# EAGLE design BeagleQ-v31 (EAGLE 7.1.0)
BOARD_NUMBER: 1.0
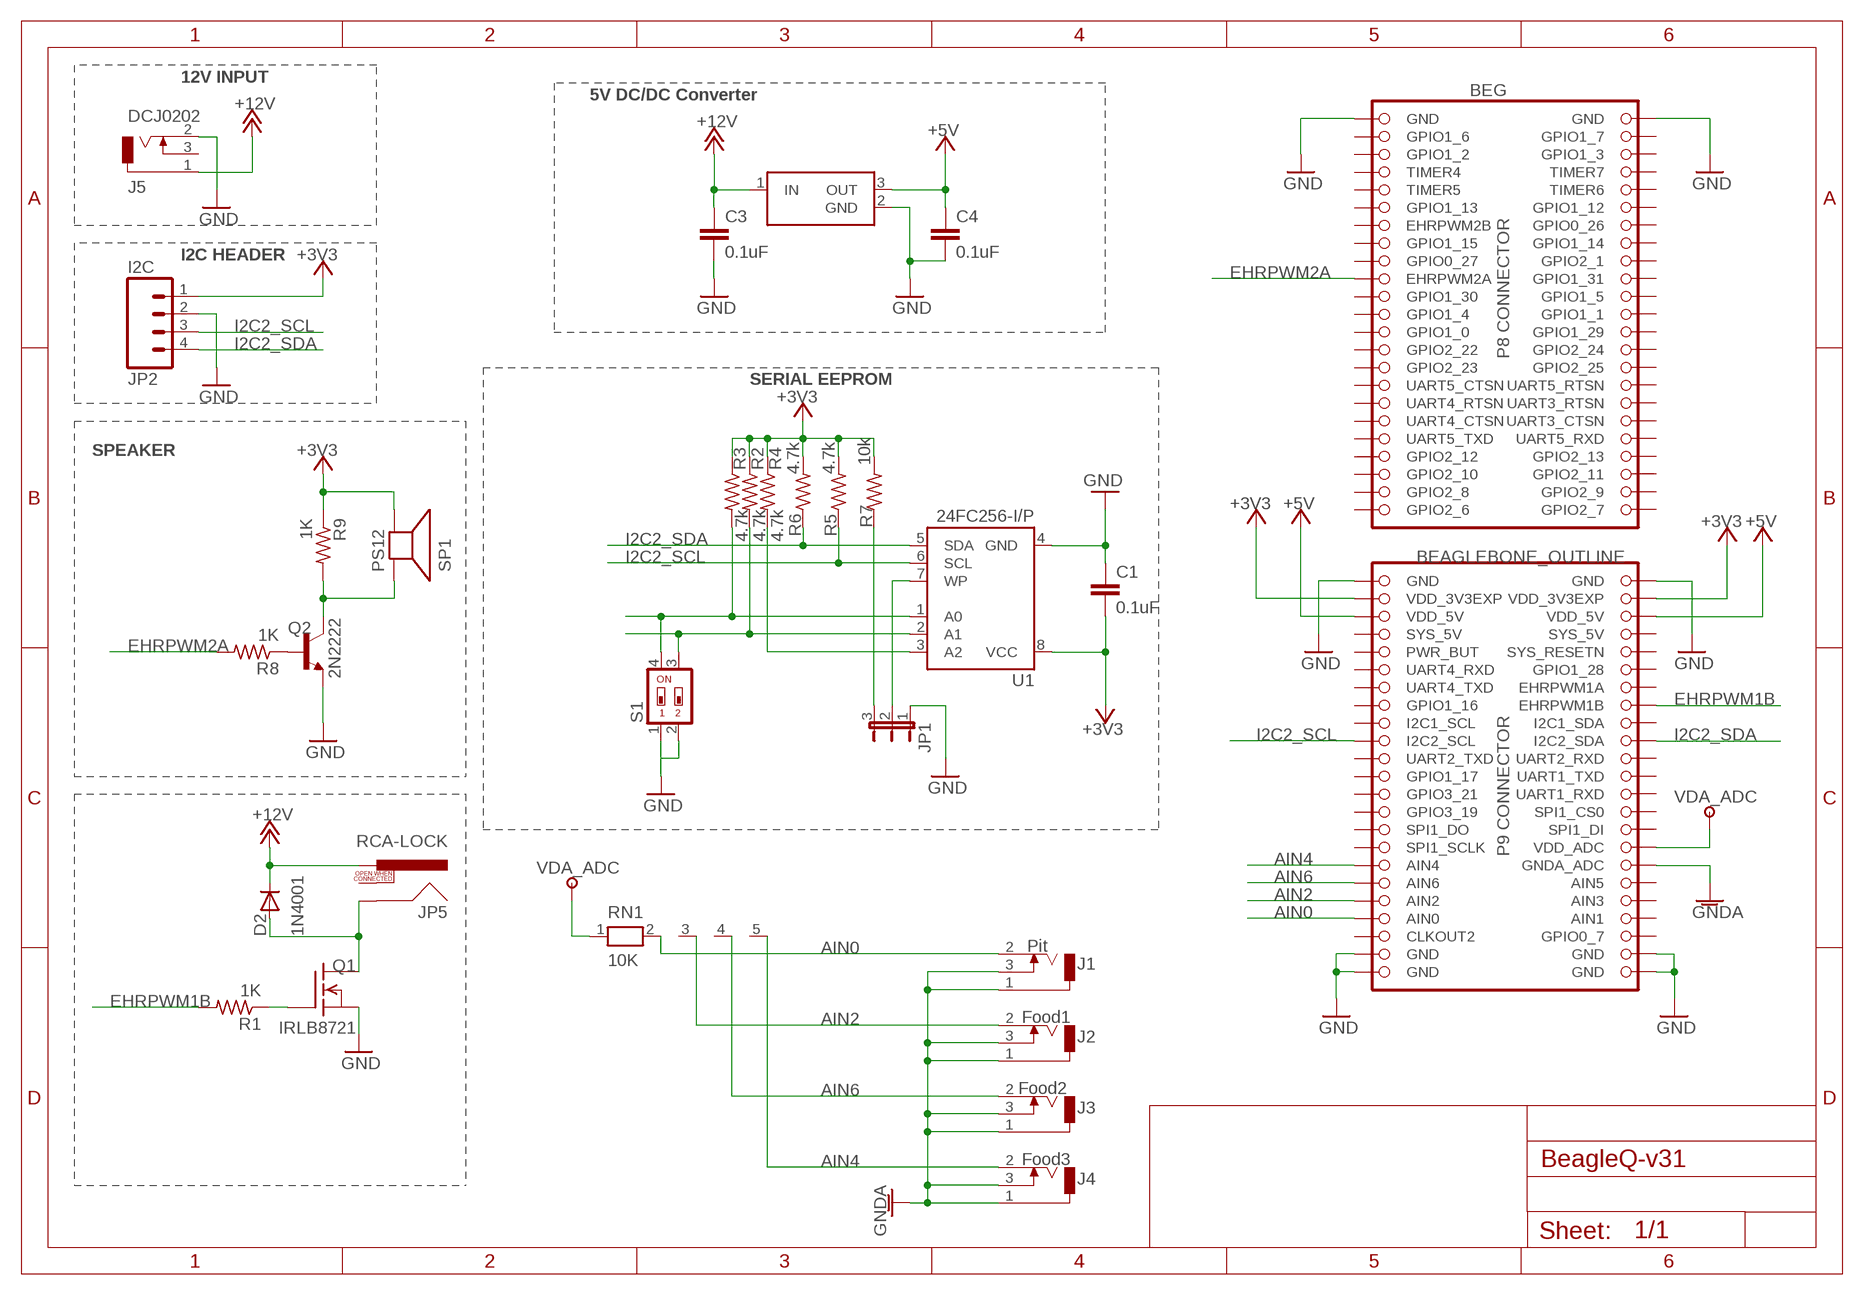
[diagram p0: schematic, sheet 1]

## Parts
BEG  BEAGLEBONE_OUTLINE  [BEAGLEBONE_SHIELD]
C1  0.1uF  C2.5/2  [C2.5-2]
C3  0.1uF  C2.5/2  [C2.5-2]
C4  0.1uF  C2.5/2  [C2.5-2]
D2  1N4001  1N4004  [DO41-10]
J1  Pit  MJ-2508N  [MJ-2508N]
J2  Food1  MJ-2508N  [MJ-2508N]
J3  Food2  MJ-2508N  [MJ-2508N]
J4  Food3  MJ-2508N  [MJ-2508N]
J5  DCJ0202  [DCJ0202]
JP1  WP  JP2E  [JP2]
JP2  I2C  M04PTH  [1X04]
JP5  RCA-LOCK  [RCA_LOCK]
Q1  IRLB8721  BUZ10  [TO220]
Q2  2N2222  [TO-92]
R1  1K  R-US_0207/10  [0207/10]
R2  4.7k  R-US_0207/10  [0207/10]
R3  4.7k  R-US_0207/10  [0207/10]
R4  4.7k  R-US_0207/10  [0207/10]
R5  4.7k  R-US_0207/10  [0207/10]
R6  4.7k  R-US_0207/10  [0207/10]
R7  10k  R-US_0207/10  [0207/10]
R8  1K  R-US_0207/10  [0207/10]
R9  1K  R-US_0207/10  [0207/10]
RN1  10K  RN04  [RN-5]
S1  SWS002  [SMS-002]
SP1  PS12  SPEAKER/PS12  [PS12]
U1  24FC256-I/P  AT24CP  [DIL08]
U2  OKI-78SRHZNTL  [OKI-78SR-HZNTL]

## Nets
+3V3: BEG.49(VDD_3V3EXP) BEG.50(VDD_3V3EXP) C1.2 JP2.1 R2.1 R3.1 R4.1 R5.2 R6.2 R7.2 R9.1 SP1.P$2(-) U1.8(VCC)
+5V [VDD]: BEG.51(VDD_5V) BEG.52(VDD_5V) C4.1 U2.3(OUT)
+12V: C3.1 D2.C J5.1 JP5.PIN U2.1(IN)
AIN0: BEG.85(AIN0) J1.2 RN1.2
AIN2: BEG.83(AIN2) J2.2 RN1.3
AIN4: BEG.79(AIN4) J4.2 RN1.5
AIN6: BEG.81(AIN6) J3.2 RN1.4
BLOWER_L [VCC_12V]: D2.A JP5.SHELL Q1.2(D)
EHRPWM1B: BEG.62(EHRPWM1B) R1.2
EHRPWM2A: BEG.19(EHRPWM2A) R8.2
GND [GND]: BEG.1(GND) BEG.2(GND) BEG.47(GND) BEG.48(GND) BEG.89(GND) BEG.90(GND) BEG.91(GND) BEG.92(GND) C1.1 C3.2 C4.2 J5.2 JP1.1 JP2.2 Q1.3(S) Q1.4(S) Q2.1(E) S1.1 S1.2 U1.4(GND) U2.2(GND)
GNDA: BEG.80(GNDA_ADC) J1.1 J1.3 J2.1 J2.3 J3.1 J3.3 J4.1 J4.3
I2C2_SCL: BEG.65(I2C2_SCL) JP2.3 R5.1 U1.6(SCL)
I2C2_SDA: BEG.66(I2C2_SDA) JP2.4 R6.1 U1.5(SDA)
N$1: R2.2 S1.3 U1.2(A1)
N$2: R3.2 S1.4 U1.1(A0)
N$3: JP1.2 U1.7(WP)
N$4: Q1.1(G) R1.1
N$5: JP1.3 R7.1
N$9: R4.2 U1.3(A2)
N$12: Q2.2(B) R8.1
N$13: Q2.3(C) R9.2 SP1.P$1(+)
VDA_ADC: BEG.78(VDD_ADC) RN1.1
Unconnected: BEG.3(GPIO1_6) BEG.4(GPIO1_7) BEG.5(GPIO1_2) BEG.6(GPIO1_3) BEG.7(TIMER4) BEG.8(TIMER7) BEG.9(TIMER5) BEG.10(TIMER6) BEG.11(GPIO1_13) BEG.12(GPIO1_12) BEG.13(EHRPWM2B) BEG.14(GPIO0_26) BEG.15(GPIO1_15) BEG.16(GPIO1_14) BEG.17(GPIO0_27) BEG.18(GPIO2_1) BEG.20(GPIO1_31) BEG.21(GPIO1_30) BEG.22(GPIO1_5) BEG.23(GPIO1_4) BEG.24(GPIO1_1) BEG.25(GPIO1_0) BEG.26(GPIO1_29) BEG.27(GPIO2_22) BEG.28(GPIO2_24) BEG.29(GPIO2_23) BEG.30(GPIO2_25) BEG.31(UART5_CTSN) BEG.32(UART5_RTSN) BEG.33(UART4_RTSN) BEG.34(UART3_RTSN) BEG.35(UART4_CTSN) BEG.36(UART3_CTSN) BEG.37(UART5_TXD) BEG.38(UART5_RXD) BEG.39(GPIO2_12) BEG.40(GPIO2_13) BEG.41(GPIO2_10) BEG.42(GPIO2_11) BEG.43(GPIO2_8) BEG.44(GPIO2_9) BEG.45(GPIO2_6) BEG.46(GPIO2_7) BEG.54(SYS_5V) BEG.55(PWR_BUT) BEG.56(SYS_RESETN) BEG.57(UART4_RXD) BEG.58(GPIO1_28) BEG.59(UART4_TXD) BEG.60(EHRPWM1A) BEG.61(GPIO1_16) BEG.63(I2C1_SCL) BEG.64(I2C1_SDA) BEG.67(UART2_TXD) BEG.68(UART2_RXD) BEG.69(GPIO1_17) BEG.70(UART1_TXD) BEG.71(GPIO3_21) BEG.72(UART1_RXD) BEG.73(GPIO3_19) BEG.74(SPI1_CS0) BEG.75(SPI1_DO) BEG.76(SPI1_DI) BEG.77(SPI1_SCLK) BEG.82(AIN5) BEG.84(AIN3) BEG.86(AIN1) BEG.87(CLKOUT2) BEG.88(GPIO0_7) J5.3 JP5.SWITCH

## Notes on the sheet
- 12V INPUT
- 5V DC/DC Converter
- I2C HEADER
- SERIAL EEPROM
- SPEAKER

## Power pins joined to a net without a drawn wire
SYS_5V: BEG.53(SYS_5V)

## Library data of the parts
BEG = BeagleQ-v03:BEAGLEBONE_OUTLINE: Should match A3 pinout - but not completely tested
C1 C3 C4 = capacitor-wima:C: CAPACITOR
D2 = BeagleQ-v03:1N4004: DIODE
J1-J4 = BeagleQ-v03:MJ-2508N
J5 = BeagleQ-v03:DCJ0202: DC POWER JACK Source: DCJ0202.pdf; OC_FARNELL: unknown; OC_NEWARK: unknown
JP1 = jumper:JP2E: JUMPER
JP2 = SparkFun-Connectors:M04: Header 4 Standard 4-pin 0.1" header. Use with straight break away headers (SKU : PRT-00116), right angle break away headers (PRT-00553), swiss pins (PRT-00743), machine pins (PRT-00117), and female headers (PRT-00115). Molex polarized connector foot print use with SKU : PRT-08231 with associated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
JP5 = BeagleQ-v03:RCA
Q1 = BeagleQ-v03:BUZ10: N-Channel Enhancement MOSFET 50V; 20A; 0,080Ohm
Q2 = BeagleQ-v03:2N2222*: NPN Transistor
R1 R8 R9 = BeagleQ-v03:R-US_: RESISTOR, American symbol
R2-R7 = resistor:R-US_: RESISTOR, American symbol
RN1 = BeagleQ-v03:RN04: RESISTOR NETWORK; OC_FARNELL: unknown; OC_NEWARK: unknown
S1 = BeagleQ-v03:SWS002: SMD Dip Switch 2 pol.
SP1 = adafruit:SPEAKER: SPEAKER
U1 = BeagleQ-v03:AT24C*: 2-wire serial EEPROM; MPN: AT24C1024BW-SH-B; OC_FARNELL: 1362646; OC_NEWARK: 03P2044
U2 = BeagleQ-v03:OKI-78SR

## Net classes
0 default: width 0.203 mm
1 VCC_12V: width 0.305 mm, drill 0.406 mm
2 VDD: width 0.305 mm, drill 0.406 mm
3 GND: width 0.254 mm, drill 0.406 mm

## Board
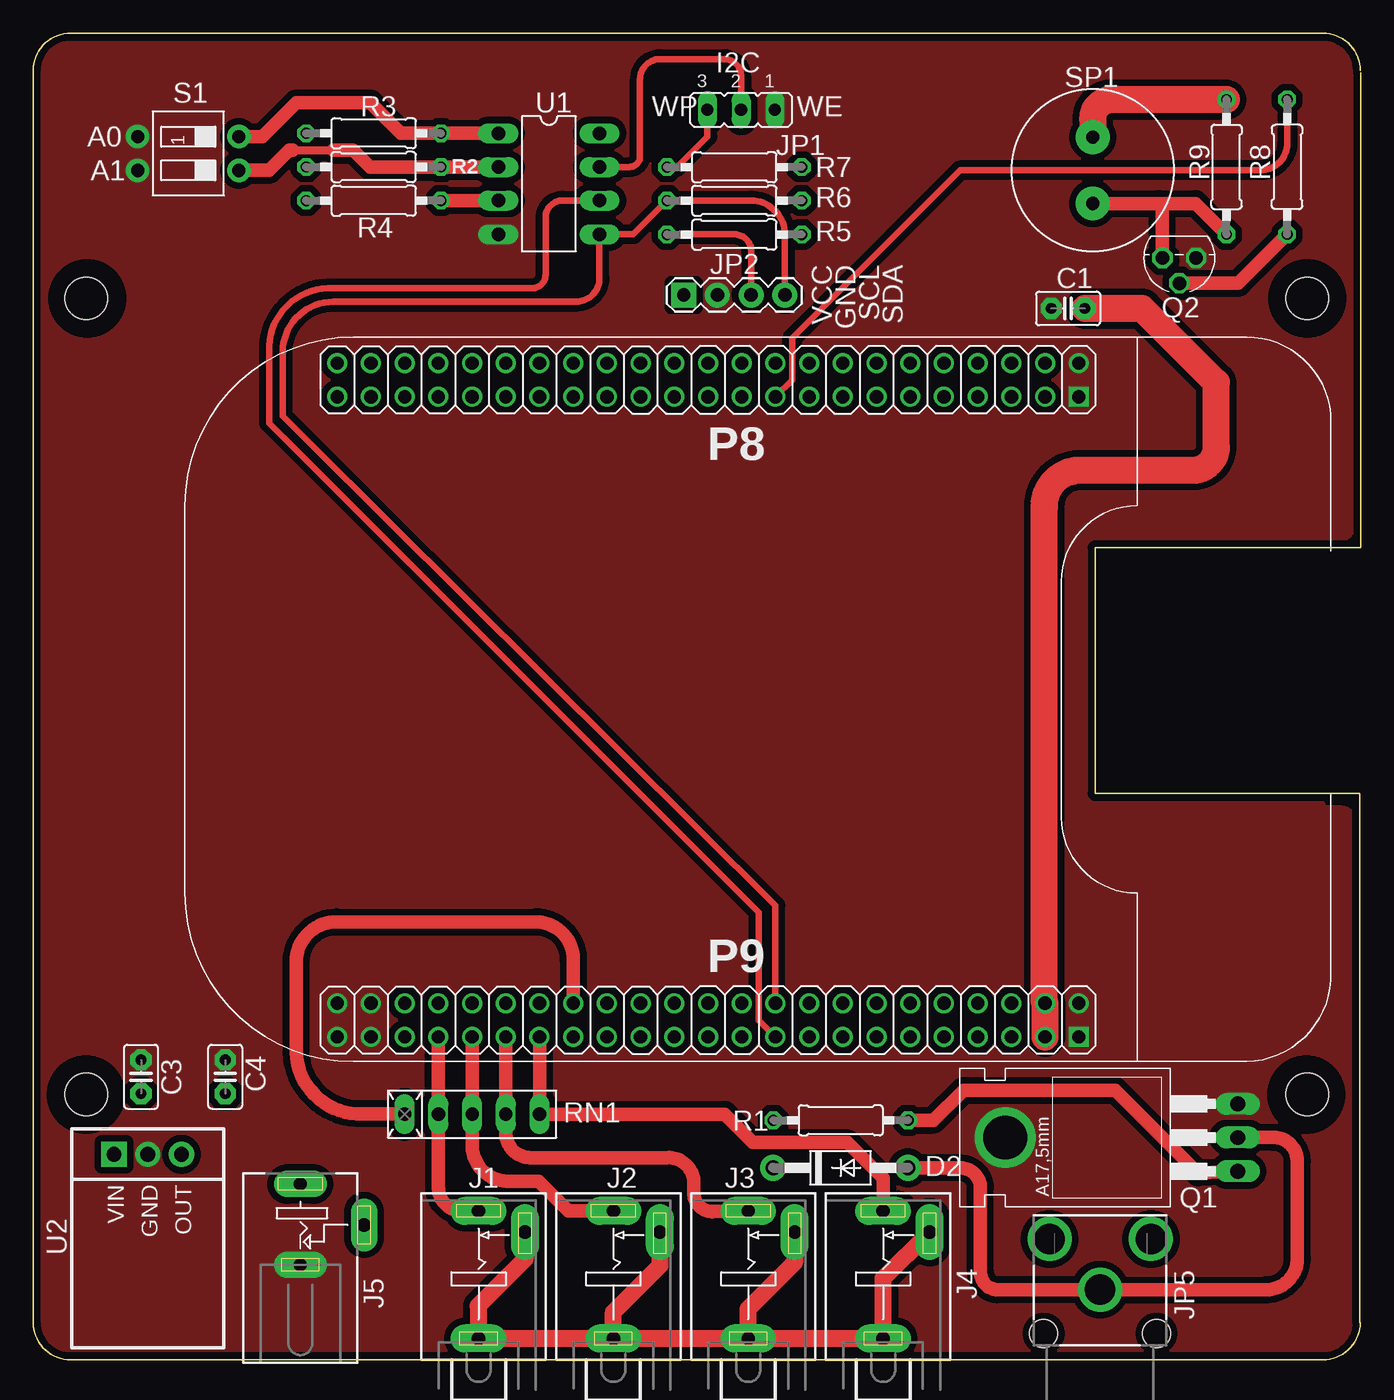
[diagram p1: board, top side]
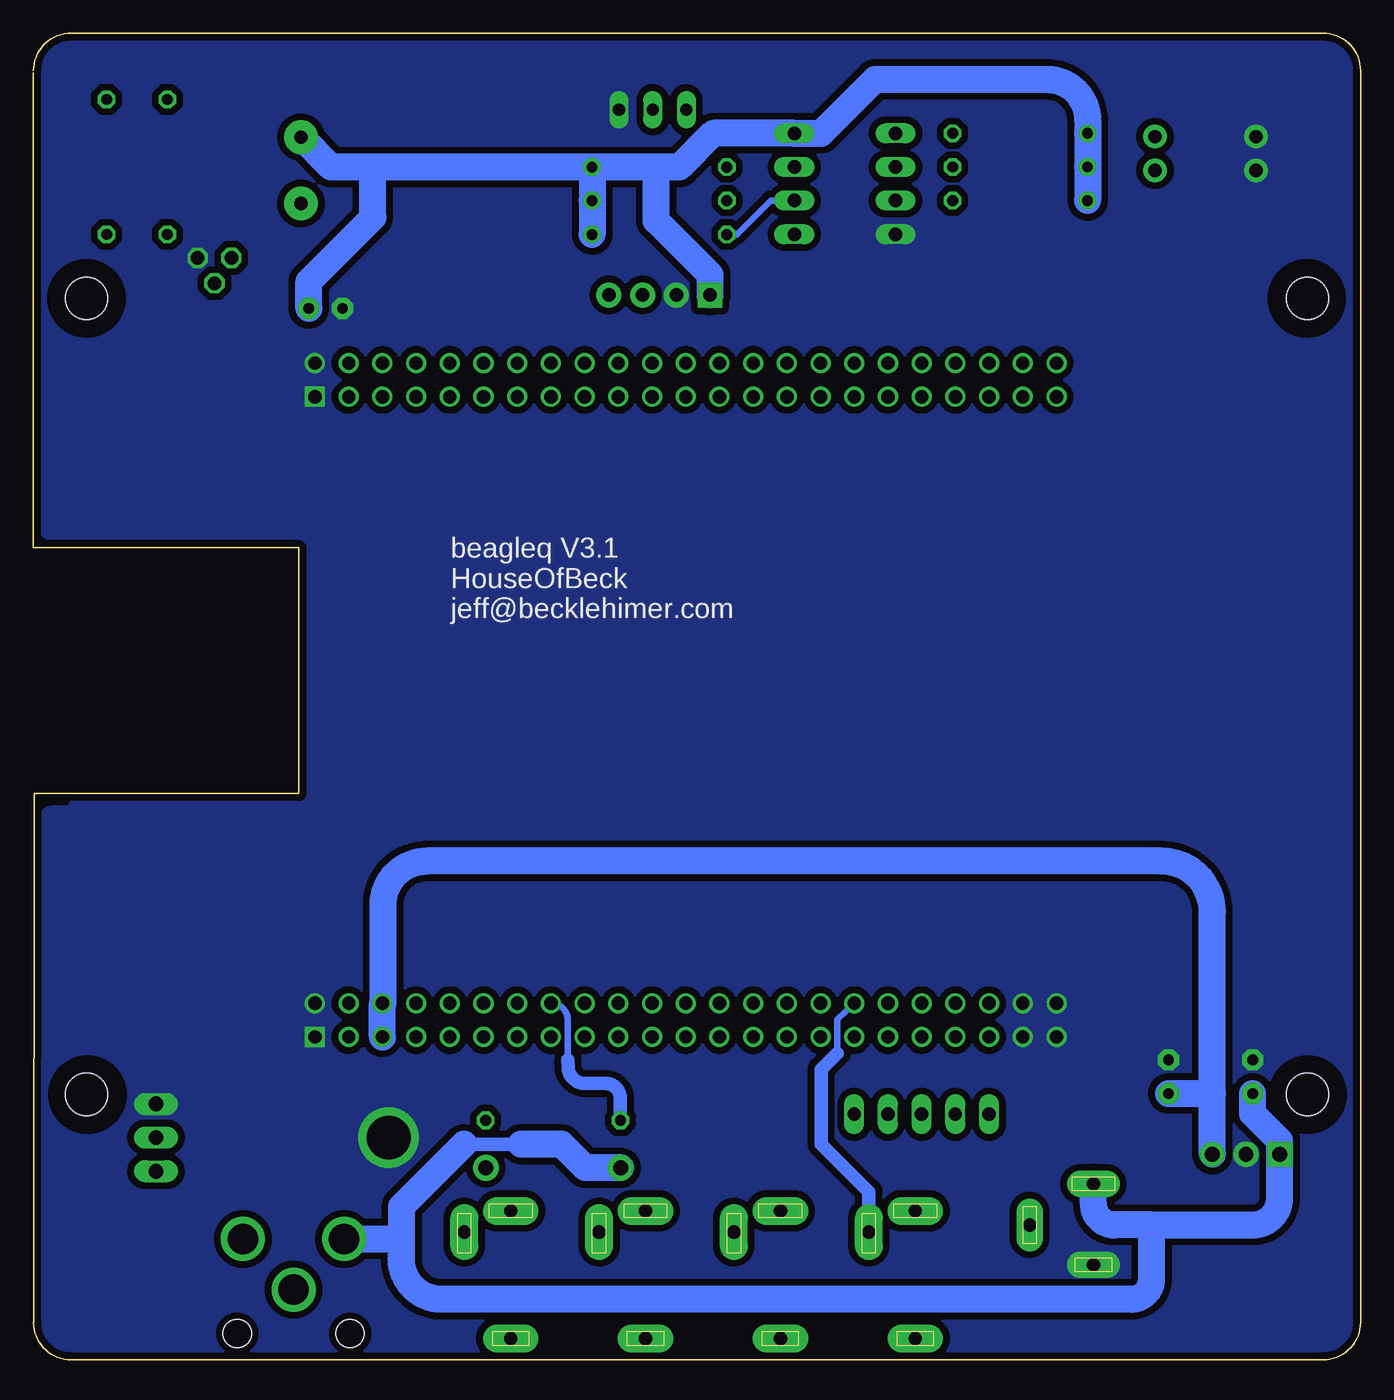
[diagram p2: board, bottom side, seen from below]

Size 100.02 x 100 mm. Coordinates in mm from the lower left corner, seen from the top.
Copper layers 1*16: Top 0.035mm / dielectric 1.5mm / Bottom 0.035mm
Design rules "dirt_cheap_dirty_boards.v1 *": minimum track width 5mil, minimum drill 12mil, track to track 10mil, track to pad 10mil, pad to pad 10mil, via to via 10mil, smd to smd 0mil, copper to edge 20mil, drill to drill 20mil, minimum pad ring 10mil, minimum via ring 6mil, stop-mask expansion 2mil, vias tented up to drill 25mil, thermal gap 10mil
tRestrict: area 93.8,77.8 to 98.2,82.2; area 1.9,77.8 to 6.2,82.2; area 1.8,17.8 to 6.2,22.2; area 93.8,17.8 to 98.1,22.2
bRestrict: area 93.8,77.8 to 98.2,82.2; area 1.9,77.8 to 6.2,82.2; area 1.8,17.8 to 6.2,22.2; area 93.8,17.8 to 98.1,22.2

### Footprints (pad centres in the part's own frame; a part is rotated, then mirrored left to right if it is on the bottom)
BEAGLEBONE_SHIELD = drill 1 square: 1 78.79,72.595; 47 78.79,24.335 | drill 1: 2 78.79,75.135; 3 76.25,72.595; 4 76.25,75.135; 5 73.71,72.595; 6 73.71,75.135; 7 71.17,72.595; 8 71.17,75.135; 9 68.63,72.595; 10 68.63,75.135; 11 66.09,72.595; 12 66.09,75.135; 13 63.55,72.595; 14 63.55,75.135; 15 61.01,72.595; 16 61.01,75.135; 17 58.47,72.595; 18 58.47,75.135; 19 55.93,72.595; 20 55.93,75.135; 21 53.39,72.595; 22 53.39,75.135; 23 50.85,72.595; 24 50.85,75.135; 25 48.31,72.595; 26 48.31,75.135; 27 45.77,72.595; 28 45.77,75.135; 29 43.23,72.595; 30 43.23,75.135; 31 40.69,72.595; 32 40.69,75.135; 33 38.15,72.595; 34 38.15,75.135; 35 35.61,72.595; 36 35.61,75.135; 37 33.07,72.595; 38 33.07,75.135; 39 30.53,72.595; 40 30.53,75.135; 41 27.99,72.595; 42 27.99,75.135; 43 25.45,72.595; 44 25.45,75.135; 45 22.91,72.595; 46 22.91,75.135; 48 78.79,26.875; 49 76.25,24.335; 50 76.25,26.875; 51 73.71,24.335; 52 73.71,26.875; 53 71.17,24.335; 54 71.17,26.875; 55 68.63,24.335; 56 68.63,26.875; 57 66.09,24.335; 58 66.09,26.875; 59 63.55,24.335; 60 63.55,26.875; 61 61.01,24.335; 62 61.01,26.875; 63 58.47,24.335; 64 58.47,26.875; 65 55.93,24.335; 66 55.93,26.875; 67 53.39,24.335; 68 53.39,26.875; 69 50.85,24.335; 70 50.85,26.875; 71 48.31,24.335; 72 48.31,26.875; 73 45.77,24.335; 74 45.77,26.875; 75 43.23,24.335; 76 43.23,26.875; 77 40.69,24.335; 78 40.69,26.875; 79 38.15,24.335; 80 38.15,26.875; 81 35.61,24.335; 82 35.61,26.875; 83 33.07,24.335; 84 33.07,26.875; 85 30.53,24.335; 86 30.53,26.875; 87 27.99,24.335; 88 27.99,26.875; 89 25.45,24.335; 90 25.45,26.875; 91 22.91,24.335; 92 22.91,26.875 | hole 3.2: 4,80; 96,80; 96,20; 4,20
C2.5-2 = drill 0.813 pad 1.6 octagon: 1 -1.27,0; 2 1.27,0
DO41-10 = drill 1.118 pad 1.93: A 5.08,0; C -5.08,0
MJ-2508N = drill 1 pad 2.1 long: 1 0,-6.52; 2 0,3.1; 3 3.5,1.5
DCJ0202 = drill 1 pad 2 long: 1 0,3.1; 2 0,-3; 3 4.8,0
JP2 = drill 0.914 long: 1 -2.54,0; 2 0,0; 3 2.54,0
1X04 = drill 1.016 pad 1.88 square: 1 0,0 | drill 1.016 pad 1.88: 2 2.54,0; 3 5.08,0; 4 7.62,0
RCA_LOCK = drill 2.3: PIN 4.03,3.802; SHELL 0.203,0; SWITCH 4.03,-3.827 | hole 2.134: -3.1,4.25; -3.1,-4.25
TO220 = drill 1.118 long: 1 -2.54,-6.35; 2 0,-6.35; 3 2.54,-6.35 | drill 3.302 pad 4.572: 4 0,11.176
TO-92 = drill 1.016 octagon: 1 -1.27,0; 2 0,1.905; 3 1.27,0
0207/10 = drill 0.813 octagon: 1 -5.08,0; 2 5.08,0
RN-5 = drill 1 long: 1 -5.08,0; 2 -2.54,0; 3 0,0; 4 2.54,0; 5 5.08,0
SMS-002 = drill 1 pad 1.778: 1 -1.27,-3.81; 2 1.27,-3.81; 3 1.27,3.81; 4 -1.27,3.81
PS12 = drill 1 pad 2.54: P$1 -2.5,0; P$2 2.5,0
DIL08 = drill 1.016 long: 1 -3.81,-3.81; 2 -1.27,-3.81; 3 1.27,-3.81; 4 3.81,-3.81; 5 3.81,3.81; 6 1.27,3.81; 7 -1.27,3.81; 8 -3.81,3.81
OKI-78SR-HZNTL = drill 1.118 pad 1.905 square: 1 2.54,0 | drill 1.118 pad 1.905: 2 0,0; 3 -2.54,0

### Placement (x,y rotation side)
BEG  0,0 0 top
C1  77.98,79.25 0 top
C3  8.13,21.34 90 top
C4  14.48,21.34 90 top
D2  60.83,14.47 0 top
J1  33.56,8.13 0 top
J2  43.72,8.13 0 top
J3  53.88,8.13 0 top
J4  64.04,8.13 0 top
J5  20.13,10.16 0 top
JP1  53.34,94.23 180 top
JP2  49.02,80.26 0 top
JP5  80.39,5.08 90 top
Q1  84.42,16.75 90 top
Q2  86.36,83.06 180 top
R1  60.85,18.05 180 top
R2  25.65,89.92 0 top
R3  25.65,92.46 0 top
R4  25.65,87.38 0 top
R5  52.83,84.82 0 top
R6  52.83,87.38 0 top
R7  52.83,89.9 0 top
R8  94.49,89.92 90 top
R9  89.92,89.92 270 top
RN1  33.08,18.51 0 top
S1  11.68,90.93 270 top
SP1  79.84,89.66 90 top
U1  38.86,88.65 270 top
U2  8.64,15.49 180 top

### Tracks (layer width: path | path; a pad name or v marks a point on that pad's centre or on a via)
+3V3
  Top 2.032: BEG.49 BEG.50 arc-90 76.2,26.93 76.2,64.26 arc-90 78.74,67.06 87.38,67.06 arc90 89.15,68.83 89.15,73.66 83.57,79.25 C1.2 | R9.1 81.28,95 arc90 79.84,93.55 SP1.P$2
  Bottom 2.032: R5.2 R6.2 R7.2 | 53.34,89.92 51.31,89.92 48.77,92.46 U1.8 40.64,92.46 36.58,96.52 23.62,96.52 arc90 20.57,93.47 R3.1 R2.1 R4.1 | 53.34,89.92 57.9,89.92 R7.2 | R7.2 arc-90 57.93,89.92 74.42,89.92 | 74.42,89.92 77.59,89.92 SP1.P$2 | C1.2 79.25,81.28 74.42,86.11 74.42,89.92 | JP2.1 49.02,81.79 53.09,85.85 53.09,89.66 53.34,89.92
+5V
  Bottom 2.032: BEG.51 BEG.52 arc-90 73.66,26.93 73.66,34.29 arc90 70.36,37.59 14.99,37.59 arc90 11.18,33.78 11.18,20.07 | U2.3 11.18,20.07 | C4.1 11.18,20.07
+12V
  Top 1.016: J5.1 arc90 20.19,13.32
  Bottom 1.016: 63.25,16.26 67.56,16.26
  Bottom 2.032: D2.C 58.41,14.47 60.2,16.26 63.25,16.26 | 67.56,16.26 72.26,11.56 72.26,8.89 | 15.75,10.16 18.54,10.16 arc90 20.13,11.75 J5.1 | 15.75,10.16 15.75,6.1 arc90 17.27,4.57 69.6,4.57 arc90 72.26,8 72.26,8.89 | JP5.PIN 72.48,9.11 72.26,8.89 | 15.75,10.16 8.13,10.16 arc-90 6.1,12.19 U2.1 6.1,16.51 8.13,18.54 C3.1
AIN0
  Top 0.508: BEG.85
  Top 1.016: BEG.85 RN1.2 30.54,12.98 arc90 32.29,11.23 J1.2
AIN2
  Top 0.508: BEG.83
  Top 1.016: BEG.83 RN1.3 33.08,16.33 arc90 35.69,13.46 38.1,13.46 40.33,11.23 J2.2
AIN4
  Top 0.508: BEG.79
  Top 1.016: BEG.79 RN1.5 52.1,18.51 54.23,16.38 61.34,16.38 64.04,13.68 J4.2
AIN6
  Top 0.508: BEG.81
  Top 1.016: BEG.81 RN1.4 35.62,17.09 arc90 37.47,15.24 47.75,15.24 arc-90 49.78,13.46 49.78,12.45 arc90 51.31,11.18 53.83,11.18 arc90 J3.2
BLOWER_L
  Top 1.016: D2.A 69.86,14.47 arc-90 71.37,12.95 71.37,6.6 arc90 72.69,5.28 JP5.SHELL 92.91,5.28 arc90 95.25,7.62 95.25,14.99 arc90 93.47,16.76 90.78,16.76 Q1.2
EHRPWM1B
  Bottom 0.508: 59.74,22.61 59.74,25.63 arc-90 BEG.62
  Bottom 1.016: 59.74,22.61 59.72,22.1 arc-90 58.45,20.83 56.9,20.83 arc90 55.77,19.7 R1.2
EHRPWM2A
  Top 0.508: R8.2 94.49,91.69 arc-90 92.46,89.66 69.85,89.66 57.2,77.01 57.2,73.87 BEG.19
GND
  pour Top (isolate 0.508, no thermals): 3.05,99.57 96.52,99.57 96.77,99.57 arc-90 99.57,96.77 99.57,62.99 arc-90 98.3,61.72 80.26,61.72 arc90 79.5,60.96 79.5,42.93 arc90 80.26,42.16 96.77,42.16 arc-90 97.28,41.66 98.55,41.66 arc-90 99.57,40.64 99.57,2.79 arc-90 97.28,0.51 3.05,0.51 arc-90 0.51,3.05 0.51,97.03 arc-90
  pour Bottom (isolate 0.508, no thermals): 3.05,99.57 96.77,99.57 arc-90 99.57,96.77 99.57,62.99 arc-90 98.3,61.72 80.26,61.72 arc90 79.5,60.96 79.5,42.93 arc90 80.26,42.16 96.77,42.16 arc-90 97.28,41.66 98.55,41.66 arc-90 99.57,40.64 99.57,2.79 arc-90 97.28,0.51 3.05,0.51 arc-90 0.51,3.05 0.51,97.03 arc-90
GNDA
  Top 1.27: J2.1 J1.1 33.53,1.64 33.53,4.06 37.06,7.6 J1.3 | J2.1 J3.1 | J3.1 J4.1 64.04,6.13 J4.3 | J2.1 43.72,3.59 47.24,7.11 47.24,9.6 J2.3 | J3.1 53.88,3.84 57.38,7.34 J3.3
  Bottom 0.508: 39.42,23.11 39.42,25.66 BEG.80
  Bottom 1.016: 33.53,1.64 J1.1 | J1.3 37.06,12.68 40.64,16.26 40.64,21.89 39.42,23.11
I2C2_SCL
  Top 0.508: BEG.65 54.66,25.6 54.66,33.73 17.78,70.61 17.78,76.45 arc-90 22.61,80.77 37.59,80.77 arc90 38.61,81.79 38.61,86.11 arc-90 39.88,87.38 U1.6 | R5.1 arc-90 47.77,84.84 52.83,84.84 arc-90 54.1,83.57 JP2.3
  Bottom 0.508: R5.1 47.01,84.82 44.45,87.38 U1.6
I2C2_SDA
  Top 0.508: BEG.66 55.93,34.24 20.83,69.09 18.8,71.12 18.8,75.95 arc-90 22.61,79.76 40.89,79.76 arc90 42.67,81.53 U1.5 45.21,84.84 R6.1 54.1,87.38 arc-90 56.64,84.84 JP2.4
N$1
  Top 0.61: 19.56,91.19 22.61,91.19
  Top 1.016: U1.2 R2.2 25.4,89.92 24.13,91.19 22.61,91.19 | S1.3 17.78,89.66 19.3,91.19 19.56,91.19
N$2
  Top 1.016: S1.4 17.27,92.2 19.81,94.74 25.4,94.74 27.69,92.46 R3.2 U1.1
N$3
  Top 0.508: U1.7 44.96,89.92 arc90 45.72,90.68 45.72,96.52 arc-90 47.24,98.04 52.07,98.04 arc-90 53.34,96.77 JP1.2
N$4
  Top 1.016: R1.1 67.83,18.05 70.1,20.32 81.53,20.32 87.77,14.09 Q1.1
N$5
  Top 0.508: R7.1 48.5,89.9 50.8,92.2 JP1.3
N$9
  Top 1.016: U1.3 R4.2
N$12
  Top 1.016: Q2.2 90.81,81.15 R8.1
N$13
  Top 1.016: SP1.P$1 84.84,87.16 | 84.84,87.16 87.59,87.16 R9.2 | Q2.3 85.09,86.91 84.84,87.16
VDA_ADC
  Top 1.016: RN1.1 arc90 27.96,18.54 24.38,18.54 arc-90 19.81,23.62 19.81,29.97 arc-90 22.86,33.02 37.85,33.02 arc-90 40.69,30.18 BEG.78

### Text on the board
tPlace: I2C | WP | WE | A0 | A1 | VCC | GND | SCL | SDA
bPlace: beagleq V3.1 / HouseOfBeck / jeff@becklehimer.com

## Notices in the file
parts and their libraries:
SparkFun-Connectors: Licensing: CC v3.0 Share-Alike You are welcome to use this library for commercial purposes.
